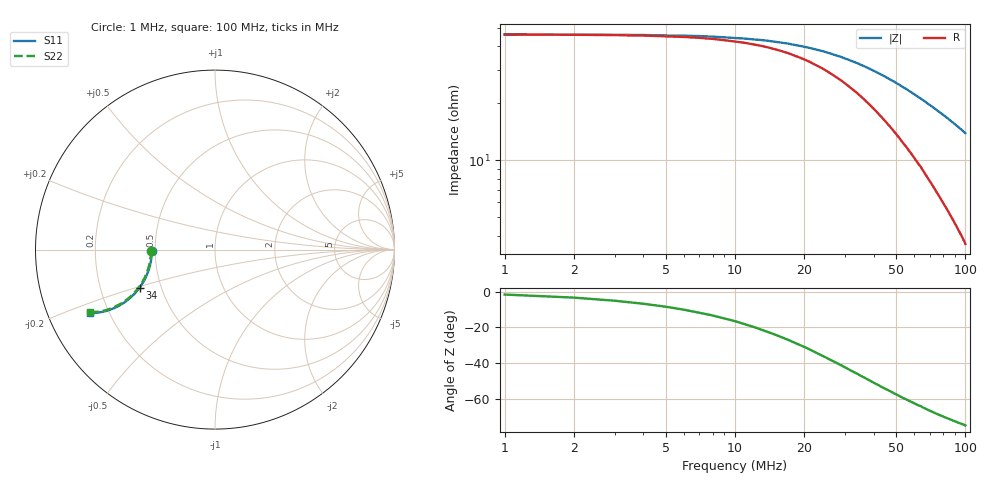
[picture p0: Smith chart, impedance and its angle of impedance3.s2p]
# Hz S RI R 50.0
! written by SimSmith version 18.3b
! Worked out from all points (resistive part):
!   100 points, 1 MHz to 100 MHz, reference 50 ohm
!   read as one part in shunt: R = 46.2 ohm at 1 MHz
!   S11 on the Smith chart (normalised r, x): 1 MHz: 0.48, -0.01; 34 MHz: 0.38, -0.21; 100 MHz: 0.13, -0.24
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1000000  -0.3514 -0.00599  0.6512 -0.00732  0.6512 -0.00732  -0.3571 -0.00616
4000000  -0.3521 -0.0278  0.6499 -0.0274  0.6499 -0.0274  -0.3574 -0.027
8000000  -0.3552 -0.0548  0.6465 -0.0537  0.6465 -0.0537  -0.3605 -0.0537
1.3e7  -0.3621 -0.0887  0.6393 -0.0868  0.6393 -0.0868  -0.3667 -0.0873
1.8e7  -0.3721 -0.121  0.6282 -0.1184  0.6282 -0.1184  -0.3769 -0.1193
2.6e7  -0.3933 -0.1693  0.6061 -0.1658  0.6061 -0.1658  -0.3976 -0.1672
3.2e7  -0.4132 -0.202  0.5846 -0.1971  0.5846 -0.1971  -0.4175 -0.2
3.4e7  -0.4204 -0.2122  0.5773 -0.206  0.5773 -0.206  -0.4243 -0.2102
4.1e7  -0.4474 -0.2452  0.5483 -0.2378  0.5483 -0.2378  -0.4514 -0.2427
4.6e7  -0.4688 -0.2659  0.5258 -0.2567  0.5258 -0.2567  -0.4728 -0.263
5.1e7  -0.4902 -0.2834  0.5028 -0.2732  0.5028 -0.2732  -0.4942 -0.2806
5.4e7  -0.5038 -0.2935  0.4885 -0.2823  0.4885 -0.2823  -0.5076 -0.2904
6.1e7  -0.535 -0.3128  0.4552 -0.2988  0.4552 -0.2988  -0.5386 -0.3092
6.3e7  -0.544 -0.3175  0.4461 -0.3026  0.4461 -0.3026  -0.5475 -0.3138
6.4e7  -0.5448 -0.3168  0.4388 -0.3026  0.4388 -0.3026  -0.5483 -0.313
6.5e7  -0.5531 -0.3219  0.4364 -0.3064  0.4364 -0.3064  -0.5566 -0.3182
6.7e7  -0.5616 -0.3263  0.4268 -0.3095  0.4268 -0.3095  -0.5649 -0.3225
6.9e7  -0.5713 -0.3298  0.4171 -0.313  0.4171 -0.313  -0.5747 -0.3258
7.7e7  -0.6056 -0.3417  0.3808 -0.3217  0.3808 -0.3217  -0.6084 -0.3373
8.4e7  -0.6343 -0.3483  0.3502 -0.325  0.3502 -0.325  -0.6366 -0.3435
9.3e7  -0.67 -0.3531  0.3127 -0.3255  0.3127 -0.3255  -0.6717 -0.348
1e8  -0.6965 -0.3537  0.285 -0.3233  0.285 -0.3233  -0.6976 -0.3486
